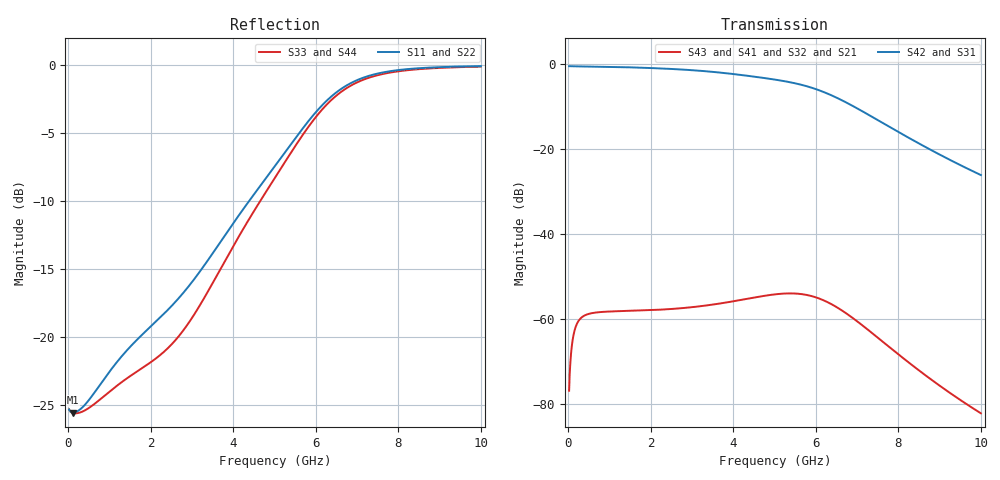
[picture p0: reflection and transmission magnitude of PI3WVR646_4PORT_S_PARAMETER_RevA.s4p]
! NPort=4 DATA=1500 NOISE=0 GROUPDELAY=0 COMPLEX_DATAFORMAT=POLAR
! NumOfBlock=1 NumOfParam=0
! .MODEL Smodel S TSTONEFILE=PI3WVR646_4PORT_S_PARAMETER_RevA.s4p  TYPE=S
!  -- The above .MODEL line can be used for the S element in the netlist.
!  Port definition:
!  Port1 = INPUT+
!  Port2 = INPUT-
!  Port3 = OUTPUT+
!  Port4 = OUTPUT-
# Hz S MA R  50
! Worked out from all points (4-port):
!   1500 points, 25 MHz to 10 GHz, reference 50 ohm
!   strongest paths, dB at 25 MHz, 2.52 GHz, 5.016 GHz, 7.511 GHz, 10 GHz:
!     S42: -0.5, -1.2, -3.7, -13.3, -26.1
!     S31: -0.5, -1.2, -3.7, -13.3, -26.1
!     S43: -76.8, -57.6, -54.2, -64.4, -82.1
!     S41: -76.8, -57.6, -54.2, -64.5, -82.2
!     S32: -76.8, -57.6, -54.2, -64.5, -82.2
!     S21: -76.8, -57.6, -54.2, -64.5, -82.3
!   lowest |S11| = -25.6 dB at 118.2 MHz (marker M1), VSWR 1.11, Z = 55.4 - j1.5 ohm
!   |S11| at or under -10 dB: start of sweep to 4.382 GHz
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2.5e7  0.05418 -4.7  0.0001444 82.4  0.9403 -1.0  0.0001444 82.4
       0.0001444 82.4  0.05418 -4.7  0.0001444 82.4  0.9403 -1.0
       0.9403 -1.0  0.0001444 82.4  0.05421 -4.3  0.0001444 82.4
       0.0001444 82.4  0.9403 -1.0  0.0001444 82.4  0.05421 -4.3
1.18162e8  0.05276 -14.8  0.0006012 57.4  0.9374 -4.4  0.0006013 57.4
           0.0006012 57.4  0.05276 -14.8  0.0006013 57.4  0.9374 -4.4
           0.9375 -4.4  0.0006013 57.4  0.05254 -12.8  0.0006013 57.4
           0.0006013 57.4  0.9375 -4.4  0.0006013 57.4  0.05254 -12.8
2.22096e9  0.1177 -174.2  0.00129 -67.7  0.885 -81.1  0.001291 -67.5
           0.00129 -67.7  0.1177 -174.2  0.001291 -67.5  0.885 -81.1
           0.8851 -81.1  0.001292 -67.5  0.08564 -169.5  0.001293 -67.3
           0.001292 -67.5  0.8851 -81.1  0.001293 -67.3  0.08564 -169.5
4.21729e9  0.2919 73.9  0.001683 -145.8  0.7382 -159.1  0.001688 -145.5
           0.001683 -145.8  0.2919 73.9  0.001688 -145.5  0.7382 -159.1
           0.7383 -159.1  0.001688 -145.4  0.2462 73.6  0.001694 -145.1
           0.001688 -145.4  0.7383 -159.1  0.001694 -145.1  0.2462 73.6
5.68127e9  0.5847 21.4  0.001943 122.7  0.5633 136.9  0.001953 123.0
           0.001943 122.7  0.5847 21.4  0.001953 123.0  0.5633 136.9
           0.5634 136.9  0.001954 123.1  0.5535 22.3  0.001964 123.4
           0.001954 123.1  0.5634 136.9  0.001964 123.4  0.5535 22.3
6.80587e9  0.8528 -17.4  0.001097 39.6  0.3382 84.8  0.001103 40.0
           0.001097 39.6  0.8528 -17.4  0.001103 40.0  0.3382 84.8
           0.3383 84.8  0.001104 40.0  0.8344 -16.9  0.001111 40.3
           0.001104 40.0  0.3383 84.8  0.001111 40.3  0.8344 -16.9
1e10  0.9924 -81.3  7.711e-05 -65.8  0.04938 9.3  7.771e-05 -65.4
      7.711e-05 -65.8  0.9924 -81.3  7.771e-05 -65.4  0.04938 9.3
      0.04939 9.4  7.774e-05 -65.4  0.9885 -81.2  7.835e-05 -65.0
      7.774e-05 -65.4  0.04939 9.4  7.835e-05 -65.0  0.9885 -81.2
